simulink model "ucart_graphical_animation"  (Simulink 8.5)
settings: Solver=ode45  StartTime=0.0  StopTime=10.0  RelTol=1e-3
libraries: vrlib x1, simulink x1

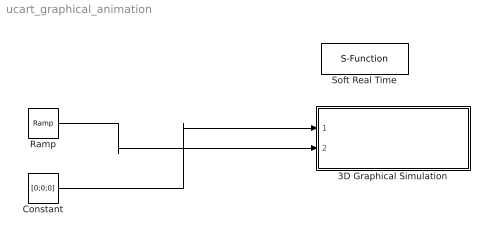
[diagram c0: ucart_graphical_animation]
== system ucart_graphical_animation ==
  3D Graphical Simulation : Subsystem
  Constant : Constant  Value=[0;0;0]
  Ramp : simulink/Sources/Ramp  slope=[ 1 ; 0 ; 0 ]  start=0  X0=0
  Soft Real Time : S-Function  FunctionName=sfun_time  Parameters=x
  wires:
  Constant/1 -> 3D Graphical Simulation/1(Displacement)
  Ramp/1 -> 3D Graphical Simulation/2(Euler Angles)

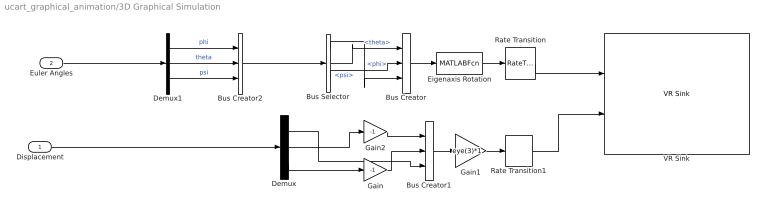
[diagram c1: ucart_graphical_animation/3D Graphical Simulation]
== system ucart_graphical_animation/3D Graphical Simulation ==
  Displacement : Inport
  Euler Angles : Inport  Port=2
  Bus Creator : BusCreator  Inputs=3
  Bus Creator1 : BusCreator  Inputs=3
  Bus Creator2 : BusCreator  Inputs=3
  Bus Selector : BusSelector  OutputSignals=phi,theta,psi
  Demux : Demux  Outputs=3
  Demux1 : Demux  Outputs=3
  Eigenaxis Rotation : MATLABFcn  MATLABFcn=eigenaxis_ucart  Output1D=off
  Gain : Gain  Gain=-1
  Gain1 : Gain  Gain=eye(3)*1  Multiplication=Matrix(K*u)
  Gain2 : Gain  Gain=-1
  Rate Transition : RateTransition  OutPortSampleTime=0.06
  Rate Transition1 : RateTransition  OutPortSampleTime=0.06
  VR Sink : vrlib/VR Sink  InstantiateOnLoad=on  SampleTime=-1  ViewEnable=on  RemoteChange=off  RemoteView=off  FieldsWritten=Helicopter.rotation.4.1.1.double#Helicopter.translation.3.1.1.double  WorldFileName=quadrotor_world_ucart.wrl  AutoView=on  VideoDimensions=[]  AllowVariableSize=off
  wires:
  Euler Angles/1 -> Demux1/1
  Displacement/1 -> Demux/1
  Bus Creator2/1 -> Bus Selector/1
  Demux/1 -> Bus Creator1/3
  Gain/1 -> Bus Creator1/2
  Gain2/1 -> Bus Creator1/1
  Rate Transition1/1 -> VR Sink/2
  Rate Transition/1 -> VR Sink/1
  Demux/3 -> Gain/1
  Demux/2 -> Gain2/1
  Bus Creator1/1 -> Gain1/1
  Bus Selector/1 -> Bus Creator/3  "<phi>"
  Bus Selector/3 -> Bus Creator/2  "<psi>"
  Bus Selector/2 -> Bus Creator/1  "<theta>"
  Bus Creator/1 -> Eigenaxis Rotation/1
  Gain1/1 -> Rate Transition1/1
  Eigenaxis Rotation/1 -> Rate Transition/1
  Demux1/3 -> Bus Creator2/3  "psi"
  Demux1/2 -> Bus Creator2/2  "theta"
  Demux1/1 -> Bus Creator2/1  "phi"
